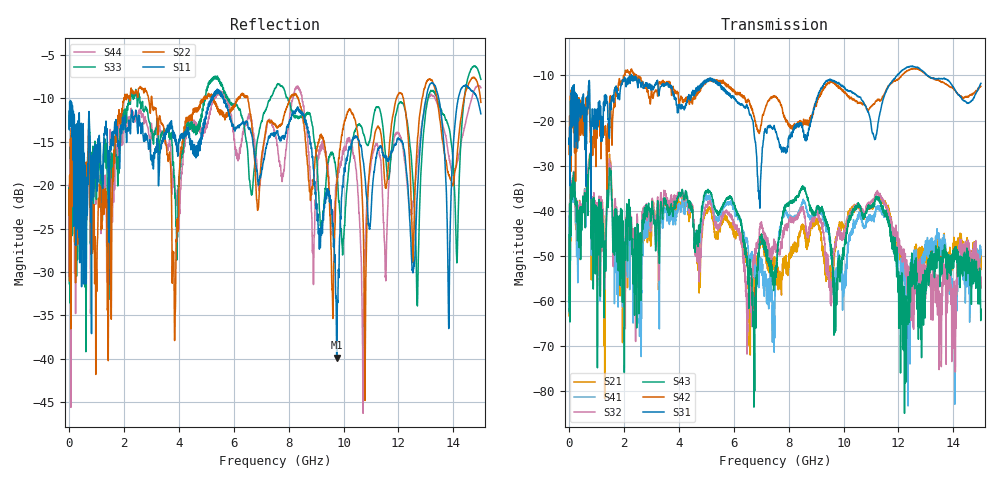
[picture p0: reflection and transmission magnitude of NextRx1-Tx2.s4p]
! FILE: N:\QM 2007\Prüfprotokolle\Highspeed\Konfektionierte Ltg\L45593-D106\D30\8216\0002\Next  Platine 2\NextRx1-Tx2.s4p
# MHz S DB R 50.00
! FREQ  S11  S12  S13  S14
!  S21  S22  S23  S24
!  S31  S32  S33  S34
!  S41  S42  S43  S44
!  DB  ANG  DB  ANG  DB  ANG  DB  ANG
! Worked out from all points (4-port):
!   2999 points, 10 MHz to 15 GHz, reference 50 ohm
!   strongest paths, dB at 10 MHz, 3.755 GHz, 7.505 GHz, 11.26 GHz, 15 GHz:
!     S31: -25.2, -12.6, -21.9, -20.6, -11.7
!     S42: -25.3, -13.4, -14.6, -15.4, -12.4
!     S43: -45.3, -40.3, -56.4, -37.3, -61.8
!     S32: -58.6, -38.2, -47.1, -36.1, -54.7
!     S41: -41.2, -42.1, -57.5, -38.9, -48.0
!     S21: -43.8, -39.9, -50.6, -36.9, -49.1
!   lowest |S11| = -39.9 dB at 9.75 GHz (marker M1), VSWR 1.02, Z = 51 - j0.154 ohm
!   |S11| at or under -10 dB: start of sweep to 5.184 GHz; 5.631 GHz to 13 GHz (7.373 GHz wide, 79.1 % of centre); 13.47 GHz to 14.18 GHz (710.6 MHz wide, 5.14 % of centre)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
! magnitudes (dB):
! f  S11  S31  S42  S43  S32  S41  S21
! 10 MHz  -11.5  -25.2  -25.3  -45.3  -58.6  -41.2  -43.8
! 730 MHz  -11.7  -11.9  -14.1  -30.7  -29.6  -29.5  -28.8
! 6.925 GHz  -19.4  -37.4  -22.9  -48.3  -46.1  -51.9  -49.5
! 9.75 GHz  -39.9  -11.5  -12.3  -60.8  -45.9  -53.1  -46.7
! 11.23 GHz  -16.2  -21.9  -15.3  -37.3  -35.5  -39.0  -37.0
! 12.22 GHz  -16.2  -8.6  -9.5  -84.9  -49.8  -54.0  -50.3
! 15 GHz  -11.8  -11.7  -12.4  -61.8  -54.7  -48.0  -49.1
